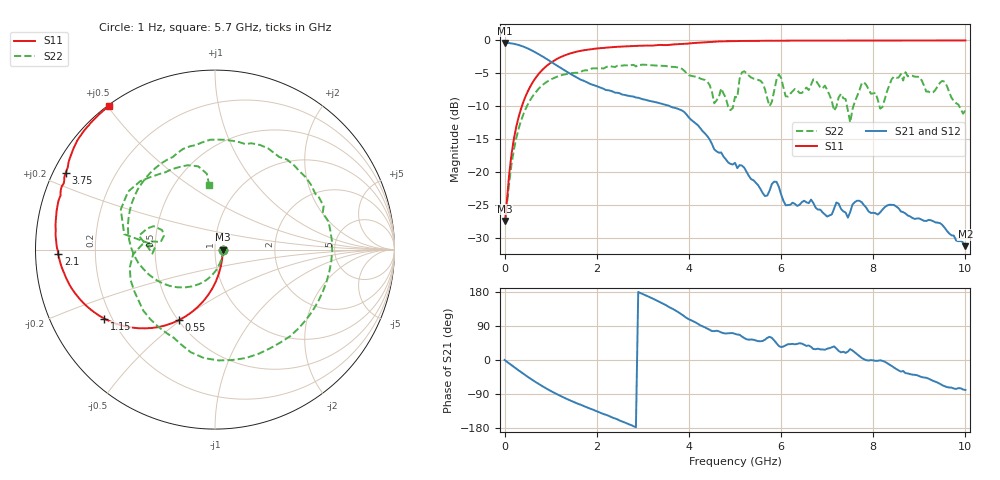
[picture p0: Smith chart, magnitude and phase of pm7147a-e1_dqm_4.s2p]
# GHz S DB R 50
! S-Parameters data
! Freq  dbS11  angS11  dbS21  angS21  dbS12  angS12  dbS22  angS22
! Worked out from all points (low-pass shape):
!   279 points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, 1 Hz to 10 GHz, reference 50 ohm
!   highest |S21| = -0.38 dB at 1.6 Hz (marker M1); lowest = -31.3 dB at 10 GHz (marker M2)
!   |S21| within 3 dB of the highest: start of sweep to 1.036 GHz
!   lowest |S11| = -27.4 dB at 1 Hz (marker M3), VSWR 1.09, Z = 54.4 - j8.75e-08 ohm
!   |S11| at or under -10 dB: start of sweep to 375.9 MHz
!   |S22| runs from -27.4 to -3.7 dB; largest |S21 - S12| = 0
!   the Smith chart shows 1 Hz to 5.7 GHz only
!   S11 on the Smith chart (normalised r, x): 1 Hz: 1.09, -0.00; 550 MHz: 0.50, -0.49; 1.15 GHz: 0.17, -0.28; 2.1 GHz: 0.07, -0.01; 3.75 GHz: 0.04, +0.24; 5.7 GHz: 0.00, +0.50
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1e-09  -27.44 -0.0  -0.38 -0.0  -0.38 -0.0  -27.44 -0.0
1.6e-09  -27.44 -0.0  -0.38 -0.0  -0.38 -0.0  -27.44 -0.0
0.2  -15.03 -88.4  -0.52 -18.2  -0.52 -18.2  -16.68 -97.4
0.55  -7.10 -117.1  -1.38 -48.4  -1.38 -48.4  -9.14 -147.7
1.15  -2.76 -148.1  -3.90 -91.1  -3.90 -91.1  -5.49 150.5
1.7  -1.52 -167.8  -6.09 -120.5  -6.09 -120.5  -4.61 107.7
2.1  -1.17 -178.4  -7.22 -140.2  -7.22 -140.2  -4.24 77.3
2.8  -0.86 167.3  -8.54 -175.0  -8.54 -175.0  -3.72 21.8
3.35  -0.70 158.4  -9.51 153.9  -9.51 153.9  -3.85 -31.8
3.75  -0.58 152.8  -10.37 127.7  -10.37 127.7  -4.11 -80.9
4.35  -0.28 144.6  -14.16 86.0  -14.16 86.0  -6.02 -160.2
5.05  -0.10 134.6  -19.42 67.3  -19.42 67.3  -8.66 174.5
5.25  -0.08 132.1  -19.96 54.8  -19.96 54.8  -4.97 137.4
5.7  -0.05 126.4  -23.59 58.4  -23.59 58.4  -8.81 95.2
6.7  -0.04 115.8  -24.71 29.0  -24.71 29.0  -5.92 75.7
7.5  -0.03 108.3  -26.08 28.8  -26.08 28.8  -12.46 53.4
7.75  -0.04 106.2  -24.60 5.4  -24.60 5.4  -6.54 53.8
8.1  -0.03 103.3  -26.46 -2.0  -26.46 -2.0  -9.07 24.6
8.35  -0.03 101.3  -24.98 -12.0  -24.98 -12.0  -6.79 45.0
8.7  -0.02 98.6  -26.31 -34.6  -26.31 -34.6  -4.84 14.5
9.6  -0.02 92.2  -28.95 -71.4  -28.95 -71.4  -6.95 -47.2
10  -0.01 89.6  -31.27 -79.0  -31.27 -79.0  -10.60 -56.2
